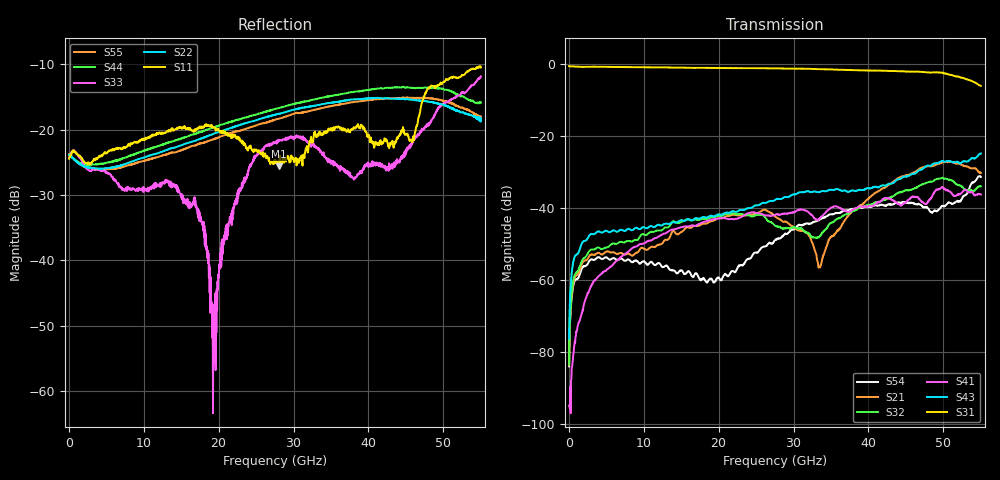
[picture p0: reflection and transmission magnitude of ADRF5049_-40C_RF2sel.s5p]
! Device  : ADRF5049
! Description: Silicon SP4T Switch Non-Reflective
! Frequency:  9kHz -  45 GHz
! Ports:
!  RFC = Port 1
!  RF1 = Port 2
!  RF2 = Port 3
!	 RF3 = Port 4
!  RF4 = Port 5
! VSS  =  +3.30 Volts
! VDD  =  -3.30 Volts
! EN  =  0.00 Volts
! LS  =  0.00 Volts
! V1  =  3.30 Volts
! V2  =  0.00 Volts
! Data:  Data was collected using an calibrated 4 port network analyzer.
! Notes: Analog Devices supplies this data as a sample of measured data
!  for this product.  Your particular data for this product may vary.
!  Data was taken at -40 degrees C.
!  Analog Devices reserves the right to change this data at anytime.
# hz S db R 50
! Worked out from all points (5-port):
!   1100 points, 50 MHz to 55 GHz, reference 50 ohm
!   strongest paths, dB at 50 MHz, 13.8 GHz, 27.55 GHz, 41.3 GHz, 55 GHz:
!     S31: -0.6, -0.9, -1.2, -1.8, -6.1
!     S43: -76.4, -44.1, -37.8, -34.3, -24.8
!     S41: -94.9, -46.0, -41.9, -38.4, -36.2
!     S32: -83.5, -43.9, -45.0, -38.2, -34.0
!     S21: -83.6, -46.6, -42.4, -35.4, -30.2
!     S54: -84.0, -57.3, -48.9, -39.3, -31.3
!   lowest |S11| = -25.6 dB at 28 GHz (marker M1), VSWR 1.11, Z = 53.1 - j4.41 ohm
!   |S11| at or under -10 dB: start of sweep to end of sweep
